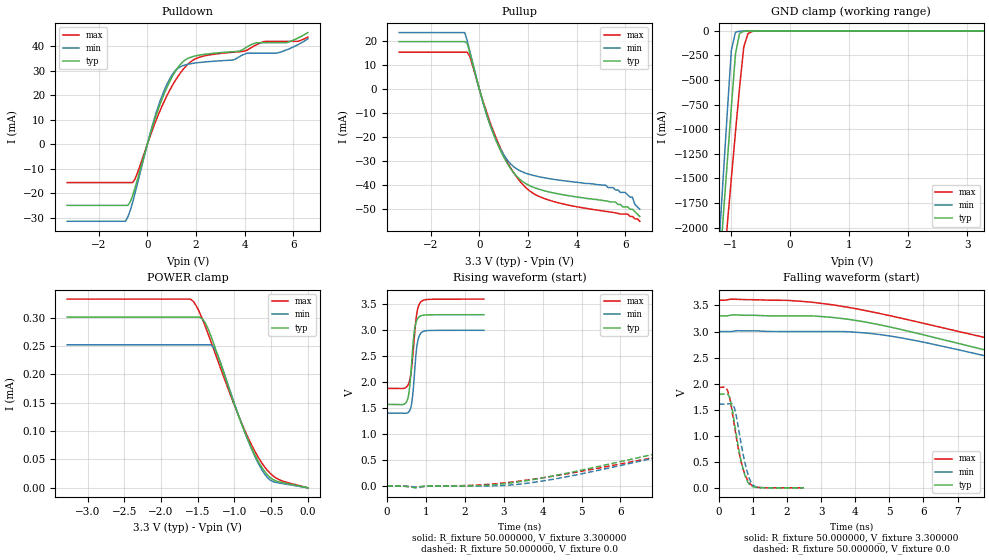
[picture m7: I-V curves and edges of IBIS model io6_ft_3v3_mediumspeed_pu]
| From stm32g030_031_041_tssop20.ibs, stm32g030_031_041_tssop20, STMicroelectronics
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|   Model io6_ft_3v3_mediumspeed_pu
[Model]  io6_ft_3v3_mediumspeed_pu
Model_type I/O
Polarity   Non-Inverting
Enable   Active-Low
Vinl =   0.990000V
Vinh =   2.310000V
Vmeas =  1.650000V
Cref =   40.000000pF
Rref =   100.000000M
Vref =   0.0V
C_comp   1.290400pF   1.272500pF   1.305600pF
[Temperature Range]   25.000000   -40.000000   0.125000k
[Pullup Reference]   3.300000V   3.000000V   3.600000V
[Pulldown Reference]   0.0V   0.0V   0.0V
[POWER Clamp Reference]   3.300000V   3.000000V   3.600000V
[GND Clamp Reference]   0.0V   0.0V   0.0V
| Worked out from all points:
|   slope of the pulldown table from 0 to 0.495 V, typ, clamps not added: 31.8 ohm
|   slope of the pullup table from 0 to 0.495 V, typ, clamps not added: 30.4 ohm
|   GND clamp passes 1 mA (typ) near -0.65 V on its own axis
|   rising waveform, R_fixture 50.000000, V_fixture 3.300000: 20-80 % time 114ps typ, 109ps min, 129ps max; typ from 1.57 V to 3.3 V
|   rising waveform, R_fixture 50.000000, V_fixture 0.0: 20-80 % time 8.24ns typ, 7.46ns min, 10.1ns max; typ from 0.002 V to 1.8 V
|   falling waveform, R_fixture 50.000000, V_fixture 3.300000: 20-80 % time 7.53ns typ, 7.46ns min, 8.06ns max; typ from 3.3 V to 1.57 V
|   falling waveform, R_fixture 50.000000, V_fixture 0.0: 20-80 % time 300ps typ, 289ps min, 332ps max; typ from 1.8 V to 0.002 V
[Pulldown]
|Voltage   I(typ)   I(min)   I(max)
-3.3V     -25.03mA   -31.54mA   -15.7mA
-900mV    -25.03mA   -31.54mA   -15.7mA
-700mV    -23.48mA   -26.95mA   -15.7mA
-500mV    -17.69mA   -19.75mA   -14.07mA
100mV     3.479mA    3.853mA    2.862mA
500mV     15.71mA    16.96mA    13.17mA
900mV     25.22mA    26.33mA    21.66mA
1.3V      31.91mA    31.32mA    28.29mA
2.2V      36.48mA    33.43mA    35.69mA
4.1V      39.76mA    37.15mA    38.42mA
5.3V      41.43mA    37.15mA    42.02mA
6.6V      45.6mA     43.04mA    43.74mA
[Pullup]
|Voltage   I(typ)   I(min)   I(max)
-3.3V     19.63mA    23.38mA    15.25mA
-600mV    19.63mA    23.38mA    15.25mA
-500mV    18.97mA    20.19mA    15.25mA
-400mV    15.37mA    16.06mA    13.73mA
100mV     -3.672mA   -3.825mA   -3.371mA
600mV     -19.12mA   -19.15mA   -18.08mA
1.2V      -31.74mA   -30.12mA   -31.25mA
1.8V      -38.62mA   -34.59mA   -39.86mA
2.9V      -42.88mA   -37.32mA   -46.32mA
5.2V      -46.5mA    -40mA      -50.9mA
6.3V      -50mA      -45mA      -53mA
6.6V      -53mA      -50mA      -55mA
[GND_clamp]
|Voltage   I(typ)   I(min)   I(max)
-3.3V     -9.61A     -9.635A    -9.699A
-1.2V     -2.493A    -2.184A    -2.958A
-1.13V    -1.917A    -1.512A    -2.469A
-1.06V    -1.345A    -845.6mA   -1.983A
-990mV    -779.8mA   -200.2mA   -1.503A
-920mV    -235.5mA   -14.18mA   -1.03A
-850mV    -26.06mA   -3.338mA   -574.2mA
-780mV    -4.499mA   -1.808mA   -166.4mA
-710mV    -1.722mA   -869.6uA   -29.45mA
-640mV    -806.7uA   -283.7uA   -6.281mA
3.28V     0A         0A         0A
[POWER_clamp]
|Voltage   I(typ)   I(min)   I(max)
-3.28V    300.8uA    252uA      332.4uA
-1.6V     300.8uA    252uA      332.4uA
-1.56V    300.8uA    252uA      328.4uA
-1.44V    297.9uA    252uA      298.3uA
-1.36V    280.4uA    252uA      271.4uA
-1.28V    252.9uA    246.9uA    243.1uA
-1.2V     222.5uA    224.3uA    214.5uA
-920mV    118.6uA    118.8uA    119.5uA
-680mV    47.6uA     44.33uA    54.63uA
-560mV    24.08uA    19.48uA    32.08uA
-480mV    14.89uA    11.29uA    21.67uA
0V        0A         0A         0A
[Ramp]
| variable   typ   min   max
dV/dt_r  1.07594/8.22573n   0.96372/7.45021n   1.14743/10.09054n
dV/dt_f  1.03164/7.51032n   0.95298/7.43871n   1.02438/8.04152n
R_load = 50.000000
[Rising Waveform]
R_fixture= 50.000000
V_fixture= 3.300000
V_fixture_min= 3.000000
V_fixture_max= 3.600000
|time   V(typ)   V(min)   V(max)
0s        1.573V     1.408V     1.883V
435.4ps   1.577V     1.404V     1.884V
510.5ps   1.637V     1.406V     1.916V
560.6ps   1.781V     1.431V     1.98V
635.6ps   2.39V      1.598V     2.299V
700.7ps   2.971V     2.107V     2.852V
760.8ps   3.184V     2.648V     3.297V
820.8ps   3.255V     2.876V     3.489V
1.026ns   3.296V     2.993V     3.592V
2.492ns   3.3V       3V         3.6V
[Rising Waveform]
R_fixture= 50.000000
V_fixture= 0.0
V_fixture_min= 0.0
V_fixture_max= 0.0
|time   V(typ)   V(min)   V(max)
0s        1.555mV    1.096mV    2.426mV
800.8ps   -17.28mV   -31.45mV   -26.85mV
2.402ns   11.72mV    2.718mV    25.26mV
3.604ns   108.6mV    56.67mV    117.9mV
10.33ns   1.126V     1.041V     1.03V
12.89ns   1.386V     1.28V      1.306V
15.62ns   1.565V     1.431V     1.526V
19.22ns   1.688V     1.532V     1.714V
23.62ns   1.753V     1.58V      1.828V
39.88ns   1.797V     1.608V     1.926V
[Falling Waveform]
R_fixture= 50.000000
V_fixture= 3.300000
V_fixture_min= 3.000000
V_fixture_max= 3.600000
|time   V(typ)   V(min)   V(max)
0s        3.3V       3V         3.6V
2.402ns   3.3V       3V         3.58V
3.363ns   3.268V     3V         3.51V
4.725ns   3.128V     2.942V     3.345V
11.29ns   2.141V     2.035V     2.428V
13.45ns   1.915V     1.794V     2.222V
15.86ns   1.773V     1.629V     2.089V
19.38ns   1.678V     1.519V     1.995V
23.7ns    1.624V     1.46V      1.94V
39.88ns   1.573V     1.408V     1.883V
[Falling Waveform]
R_fixture= 50.000000
V_fixture= 0.0
V_fixture_min= 0.0
V_fixture_max= 0.0
|time   V(typ)   V(min)   V(max)
0s        1.797V     1.608V     1.926V
255.3ps   1.797V     1.61V      1.864V
335.3ps   1.684V     1.619V     1.664V
435.4ps   1.333V     1.571V     1.272V
505.5ps   1.041V     1.395V     988.2mV
680.7ps   432.5mV    745mV      432.3mV
795.8ps   184.6mV    394.3mV    212mV
915.9ps   53.42mV    145mV      79.78mV
1.161ns   6.604mV    11.54mV    9.77mV
2.492ns   1.555mV    1.096mV    2.426mV
